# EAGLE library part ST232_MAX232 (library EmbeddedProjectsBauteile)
RS232 Transceiver
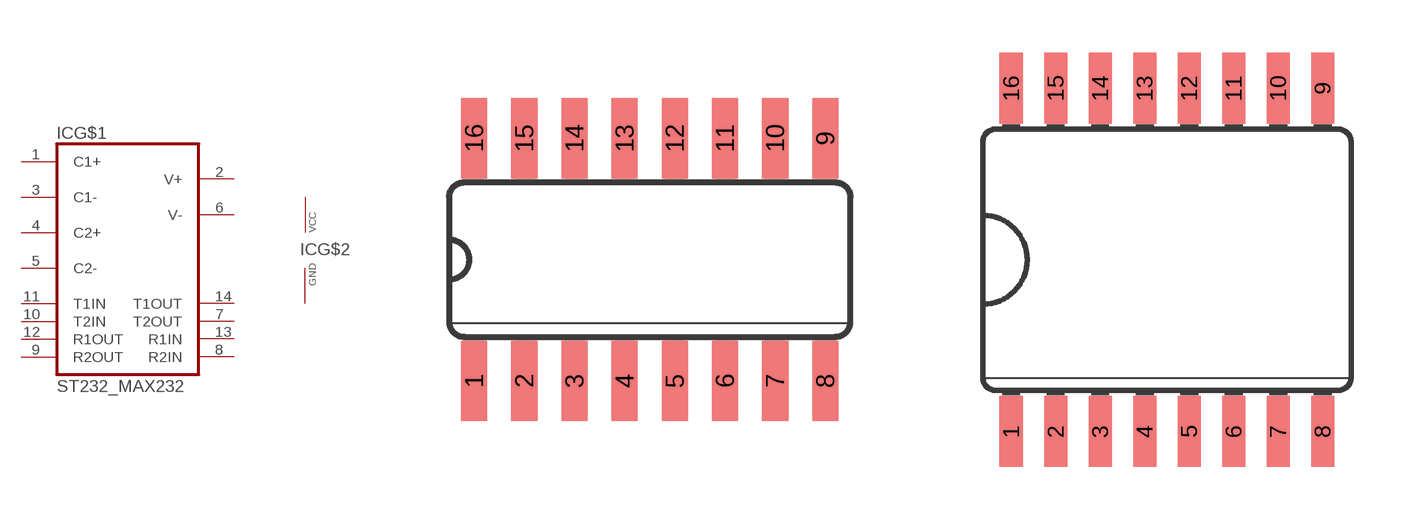
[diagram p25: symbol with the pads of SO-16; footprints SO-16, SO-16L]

Designator prefix IC; gates G$1=ST232_MAX232 G$2=VCC-GND

## ST232_MAX232D (EP: 400494)  [SO-16]
1  G$1:C1+
2  G$1:V+
3  G$1:C1-
4  G$1:C2+
5  G$1:C2-
6  G$1:V-
7  G$1:T2OUT  out
8  G$1:R2IN  in
9  G$1:R2OUT  out
10  G$1:T2IN  in
11  G$1:T1IN  in
12  G$1:R1OUT  out
13  G$1:R1IN  in
14  G$1:T1OUT  out
15  G$2:GND  pwr
16  G$2:+5V  pwr

## ST232_MAX232W  [SO-16L]
Pads as for SO-16

## Footprint SO-16 (pad centres in mm)
smd 0.66 x 2.032: 1 -4.445,-3.073; 2 -3.175,-3.073; 3 -1.905,-3.073; 4 -0.635,-3.073; 5 0.635,-3.073; 6 1.905,-3.073; 7 3.175,-3.073; 8 4.445,-3.073; 9 4.445,3.073; 10 3.175,3.073; 11 1.905,3.073; 12 0.635,3.073; 13 -0.635,3.073; 14 -1.905,3.073; 15 -3.175,3.073; 16 -4.445,3.073

## Footprint SO-16L (pad centres in mm)
smd 0.66 x 2.032: 1 -4.445,-4.902; 2 -3.175,-4.902; 3 -1.905,-4.902; 4 -0.635,-4.902; 5 0.635,-4.902; 6 1.905,-4.902; 7 3.175,-4.902; 8 4.445,-4.902; 9 4.445,4.902; 10 3.175,4.902; 11 1.905,4.902; 12 0.635,4.902; 13 -0.635,4.902; 14 -1.905,4.902; 15 -3.175,4.902; 16 -4.445,4.902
